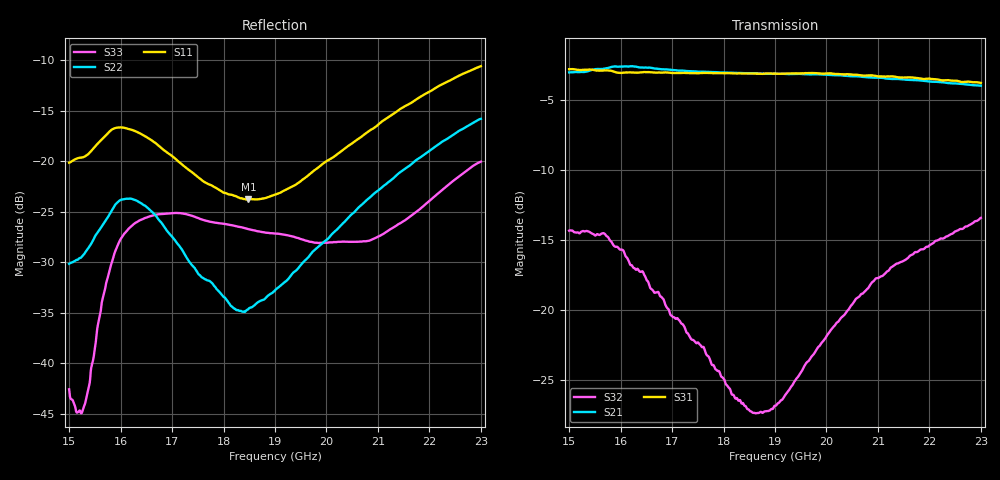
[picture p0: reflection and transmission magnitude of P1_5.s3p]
!The following data was pulled from an Agilent PNA
!This sNp file was generated from the data in the RF Test software
!NOTE:  Smoothing/Math/Corrections applied on any given trace ARE included in the data saved here
# MHz S dB R 50
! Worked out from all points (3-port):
!   1601 points, 15 GHz to 23 GHz, reference 50 ohm
!   strongest paths, dB at 15 GHz, 17 GHz, 19 GHz, 21 GHz, 23 GHz:
!     S31: -2.8, -3.1, -3.1, -3.3, -3.8
!     S21: -3.1, -2.9, -3.2, -3.4, -4.0
!     S32: -14.4, -20.4, -26.8, -17.7, -13.4
!   lowest |S11| = -23.8 dB at 18.48 GHz (marker M1), VSWR 1.14, Z = 52.5 - j6.13 ohm
!   |S11| at or under -10 dB: start of sweep to end of sweep
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15000  -20.16 51.0  -3.06 -170.0  -2.89 -169.9
       -3.05 -169.7  -30.17 83.8  -14.40 147.7
       -2.82 -169.5  -14.35 147.8  -42.60 -93.2
15605  -18.01 52.2  -2.83 -177.3  -2.99 -179.1
       -2.81 -177.4  -26.70 85.9  -14.68 133.3
       -2.92 -179.0  -14.63 133.5  -35.13 65.1
15640  -17.83 51.5  -2.80 -177.8  -3.00 -52.6
       -2.81 -177.9  -26.42 85.3  -14.63 131.6
       -2.93 -179.5  -14.55 131.9  -33.86 61.9
15680  -17.62 50.5  -2.77 -178.5  -3.00 116.2
       -2.79 -178.3  -26.12 84.9  -14.66 130.0
       -2.91 -10.7  -14.55 130.0  -33.06 57.9
15765  -17.18 47.5  -2.74 -10.7  -3.04 178.2
       -2.73 -94.7  -25.45 82.5  -14.98 126.2
       -2.91 178.5  -14.86 125.9  -31.24 52.3
15805  -16.98 45.6  -2.74 158.0  -3.08 177.6
       -2.68 74.1  -25.11 81.2  -15.17 125.1
       -2.93 177.8  -15.08 124.6  -30.42 49.0
15850  -16.82 43.0  -2.74 178.4  -3.13 177.0
       -2.65 179.0  -24.70 79.1  -15.38 123.5
       -2.98 177.0  -15.32 122.9  -29.68 45.8
18485  -23.80 -64.0  -3.20 141.0  -3.25 143.7
       -3.12 140.6  -34.65 79.5  -27.14 21.5
       -3.12 142.6  -27.11 20.8  -26.74 -57.6
19000  -23.33 -92.9  -3.18 134.1  -3.15 136.6
       -3.15 133.6  -32.80 103.9  -26.82 -14.4
       -3.14 135.5  -26.84 -15.0  -27.17 -70.6
23000  -10.60 157.3  -4.02 74.7  -3.79 76.6
       -4.00 75.2  -15.81 120.4  -13.40 -139.5
       -3.80 76.5  -13.43 -140.0  -20.05 153.3
